FUNCTION FC 100 : VOID
TITLE =GESTIONE OUTPUT
AUTHOR : MassimoZ
VERSION : 0.1

BEGIN
NETWORK
TITLE =Spia Manuale
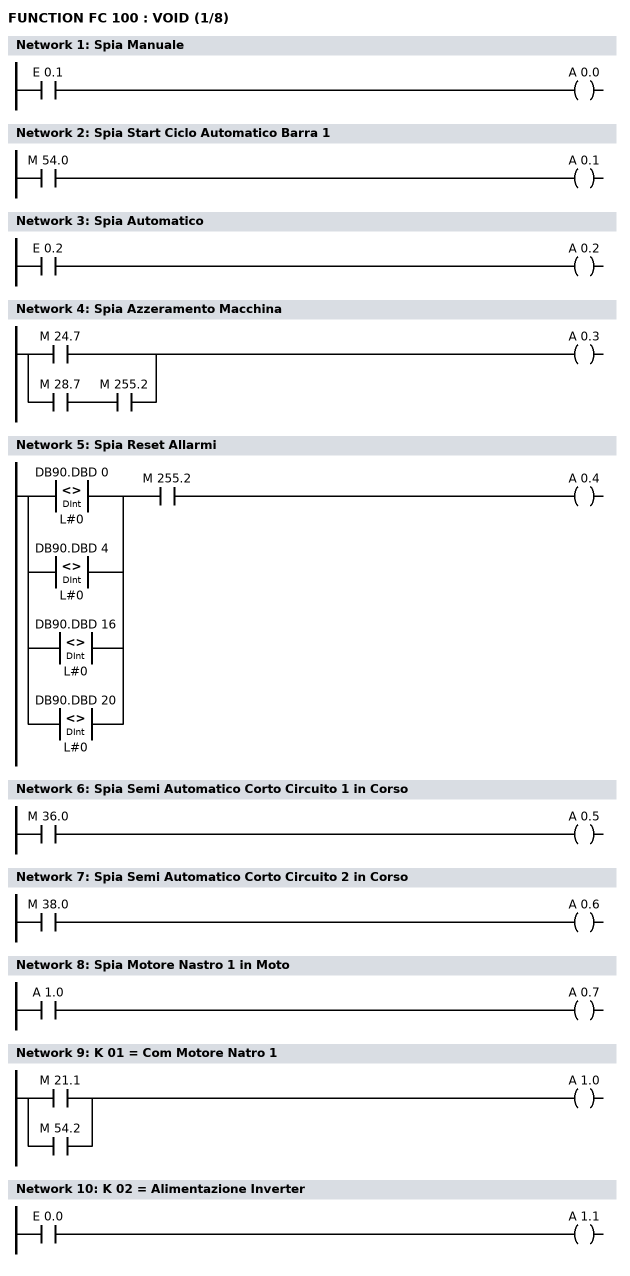
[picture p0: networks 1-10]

      U     E      0.1;
      =     A      0.0;
NETWORK
TITLE =Spia Start Ciclo Automatico Barra 1

      U     M     54.0;
      =     A      0.1;
NETWORK
TITLE =Spia Automatico

      U     E      0.2;
      =     A      0.2;
NETWORK
TITLE =Spia Azzeramento Macchina

      O     M     24.7;
      O     ;
      U     M     28.7;
      U     M    255.2;
      =     A      0.3;
NETWORK
TITLE =Spia Reset Allarmi

      U(    ;
      O(    ;
      L     DB90.DBD    0;
      L     L#0;
      <>D   ;
      )     ;
      O(    ;
      L     DB90.DBD    4;
      L     L#0;
      <>D   ;
      )     ;
      O(    ;
      L     DB90.DBD   16;
      L     L#0;
      <>D   ;
      )     ;
      O(    ;
      L     DB90.DBD   20;
      L     L#0;
      <>D   ;
      )     ;
      )     ;
      U     M    255.2;
      =     A      0.4;
NETWORK
TITLE =Spia Semi Automatico Corto Circuito 1 in Corso

      U     M     36.0;
      =     A      0.5;
NETWORK
TITLE =Spia Semi Automatico Corto Circuito 2 in Corso

      U     M     38.0;
      =     A      0.6;
NETWORK
TITLE =Spia Motore Nastro 1 in Moto

      U     A      1.0;
      =     A      0.7;
NETWORK
TITLE =K 01 = Com Motore Natro 1

      O     M     21.1;
      O     M     54.2;
      =     A      1.0;
NETWORK
TITLE =K 02 = Alimentazione Inverter

      U     E      0.0;
      =     A      1.1;
NETWORK
TITLE =K 03 = Com Motore Natro 3
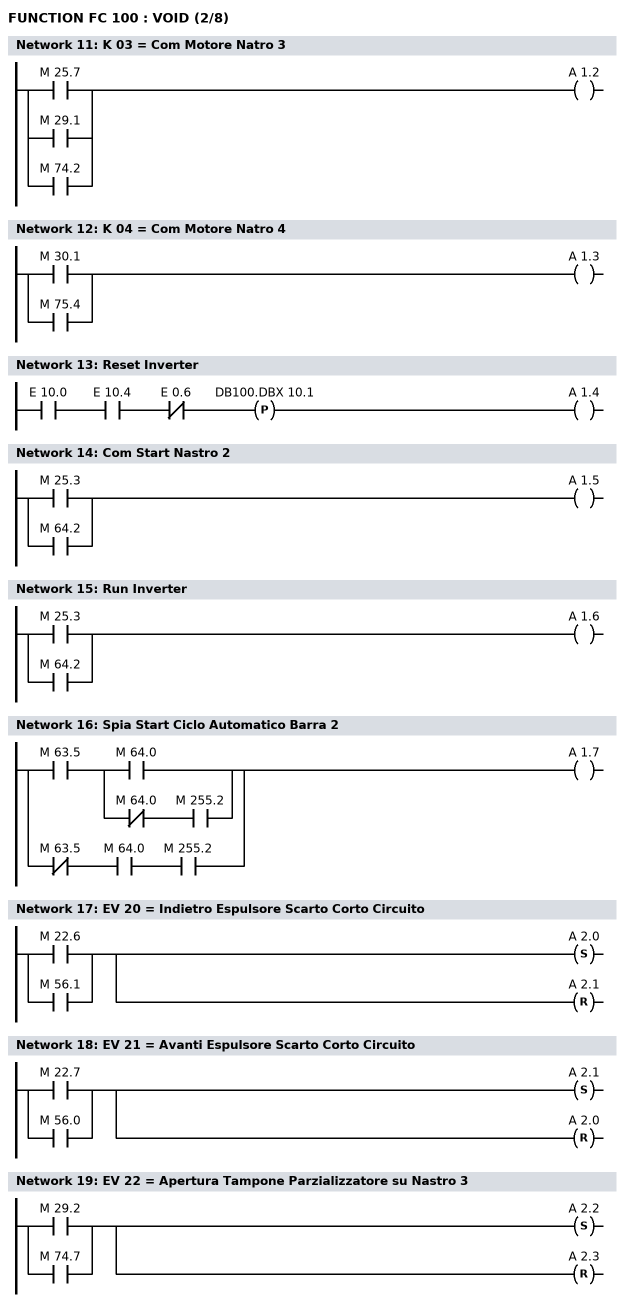
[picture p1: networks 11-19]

      O     M     25.7;
      O     M     29.1;
      O     M     74.2;
      =     A      1.2;
NETWORK
TITLE =K 04 = Com Motore Natro 4

      O     M     30.1;
      O     M     75.4;
      =     A      1.3;
NETWORK
TITLE =Reset Inverter

      U     E     10.0;
      U     E     10.4;
      UN    E      0.6;
      FP    DB100.DBX   10.1;
      =     A      1.4;
NETWORK
TITLE =Com Start Nastro 2

      O     M     25.3;
      O     M     64.2;
      =     A      1.5;
NETWORK
TITLE =Run Inverter

      O     M     25.3;
      O     M     64.2;
      =     A      1.6;
NETWORK
TITLE =Spia Start Ciclo Automatico Barra 2

      U     M     63.5;
      U(    ;
      O     M     64.0;
      O     ;
      UN    M     64.0;
      U     M    255.2;
      )     ;
      O     ;
      UN    M     63.5;
      U     M     64.0;
      U     M    255.2;
      =     A      1.7;
NETWORK
TITLE =EV 20 = Indietro Espulsore Scarto Corto Circuito

      O     M     22.6;
      O     M     56.1;
      S     A      2.0;
      R     A      2.1;
NETWORK
TITLE =EV 21 = Avanti Espulsore Scarto Corto Circuito

      O     M     22.7;
      O     M     56.0;
      S     A      2.1;
      R     A      2.0;
NETWORK
TITLE =EV 22 = Apertura Tampone Parzializzatore su Nastro 3

      O     M     29.2;
      O     M     74.7;
      S     A      2.2;
      R     A      2.3;
NETWORK
TITLE =EV 23 = Chiusura Tampone Parzializzatore su Nastro 3
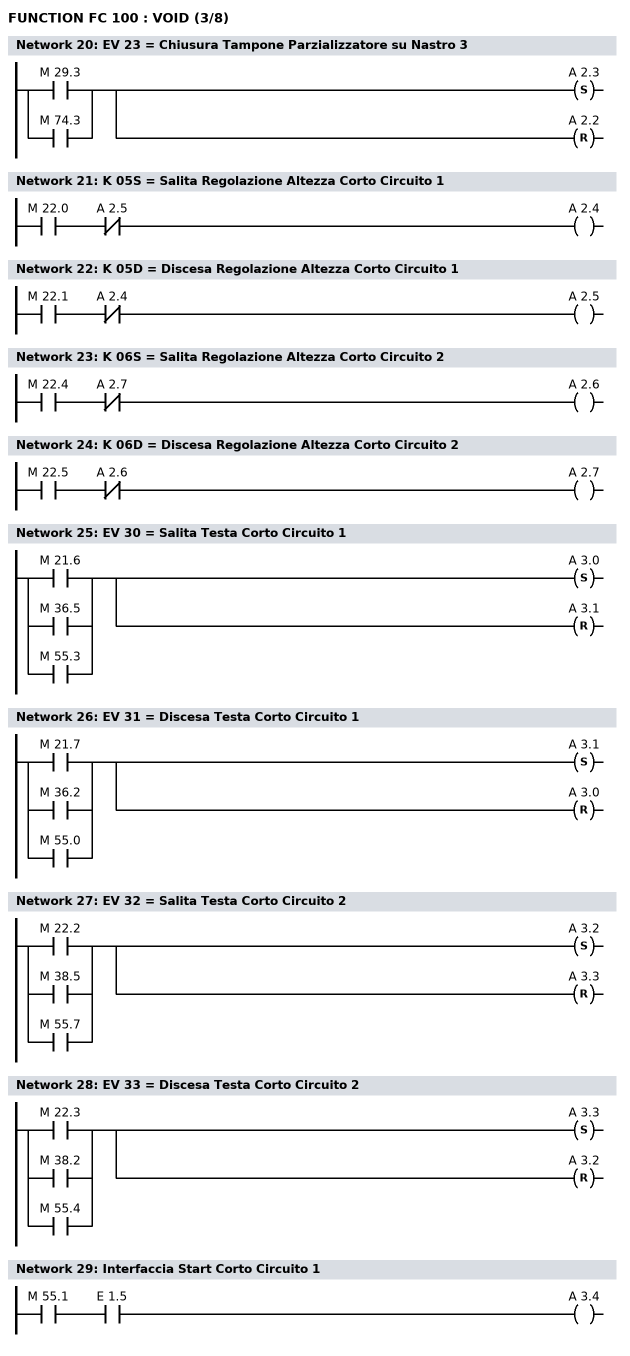
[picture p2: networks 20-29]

      O     M     29.3;
      O     M     74.3;
      S     A      2.3;
      R     A      2.2;
NETWORK
TITLE =K 05S = Salita Regolazione Altezza Corto Circuito 1

      U     M     22.0;
      UN    A      2.5;
      =     A      2.4;
NETWORK
TITLE =K 05D = Discesa Regolazione Altezza Corto Circuito 1

      U     M     22.1;
      UN    A      2.4;
      =     A      2.5;
NETWORK
TITLE =K 06S = Salita Regolazione Altezza Corto Circuito 2

      U     M     22.4;
      UN    A      2.7;
      =     A      2.6;
NETWORK
TITLE =K 06D = Discesa Regolazione Altezza Corto Circuito 2

      U     M     22.5;
      UN    A      2.6;
      =     A      2.7;
NETWORK
TITLE =EV 30 = Salita Testa Corto Circuito 1

      O     M     21.6;
      O     M     36.5;
      O     M     55.3;
      S     A      3.0;
      R     A      3.1;
NETWORK
TITLE =EV 31 = Discesa Testa Corto Circuito 1

      O     M     21.7;
      O     M     36.2;
      O     M     55.0;
      S     A      3.1;
      R     A      3.0;
NETWORK
TITLE =EV 32 = Salita Testa Corto Circuito 2

      O     M     22.2;
      O     M     38.5;
      O     M     55.7;
      S     A      3.2;
      R     A      3.3;
NETWORK
TITLE =EV 33 = Discesa Testa Corto Circuito 2

      O     M     22.3;
      O     M     38.2;
      O     M     55.4;
      S     A      3.3;
      R     A      3.2;
NETWORK
TITLE =Interfaccia Start Corto Circuito 1

      U     M     55.1;
      U     E      1.5;
      =     A      3.4;
NETWORK
TITLE =Interfaccia Start Corto Circuito 2
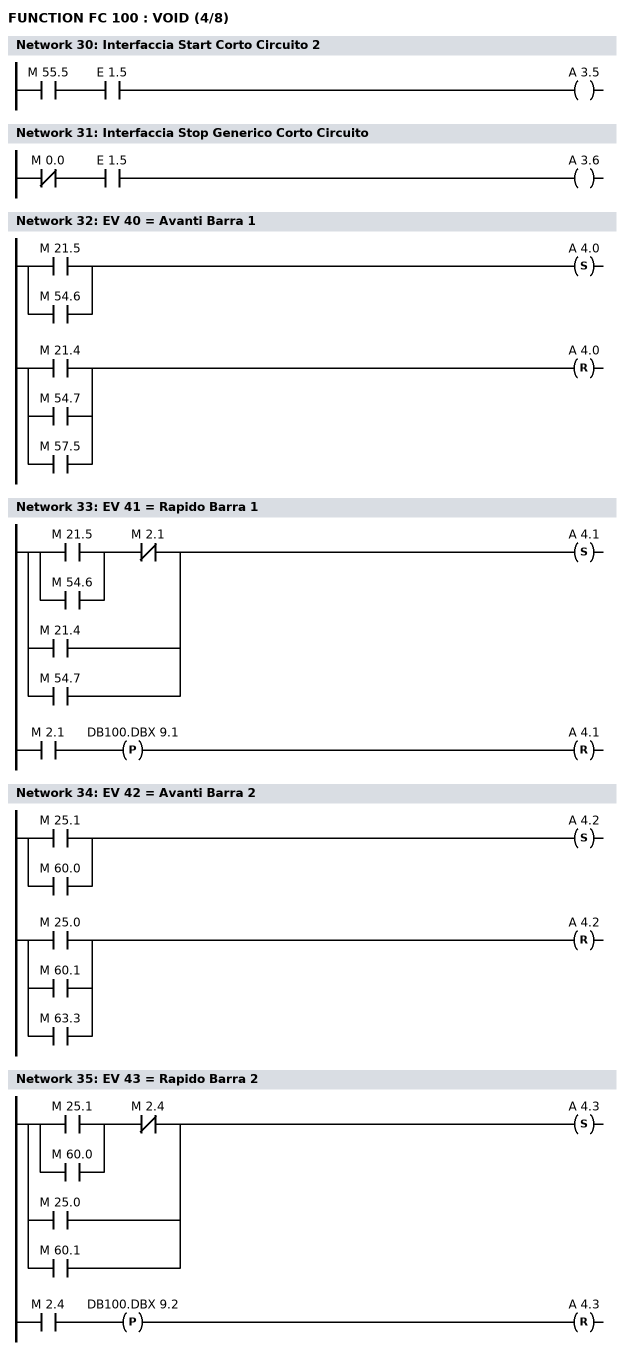
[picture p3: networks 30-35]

      U     M     55.5;
      U     E      1.5;
      =     A      3.5;
NETWORK
TITLE =Interfaccia Stop Generico Corto Circuito

      UN    M      0.0;
      U     E      1.5;
      =     A      3.6;
NETWORK
TITLE =EV 40 = Avanti Barra 1

      U(    ;
      O     M     21.5;
      O     M     54.6;
      )     ;
      S     A      4.0;
      U(    ;
      O     M     21.4;
      O     M     54.7;
      O     M     57.5;
      )     ;
      R     A      4.0;
      NOP   0;
NETWORK
TITLE =EV 41 = Rapido Barra 1

      U(    ;
      U(    ;
      O     M     21.5;
      O     M     54.6;
      )     ;
      UN    M      2.1;
      O     M     21.4;
      O     M     54.7;
      )     ;
      S     A      4.1;
      U     M      2.1;
      FP    DB100.DBX    9.1;
      R     A      4.1;
      NOP   0;
NETWORK
TITLE =EV 42 = Avanti Barra 2

      U(    ;
      O     M     25.1;
      O     M     60.0;
      )     ;
      S     A      4.2;
      U(    ;
      O     M     25.0;
      O     M     60.1;
      O     M     63.3;
      )     ;
      R     A      4.2;
      NOP   0;
NETWORK
TITLE =EV 43 = Rapido Barra 2

      U(    ;
      U(    ;
      O     M     25.1;
      O     M     60.0;
      )     ;
      UN    M      2.4;
      O     M     25.0;
      O     M     60.1;
      )     ;
      S     A      4.3;
      U     M      2.4;
      FP    DB100.DBX    9.2;
      R     A      4.3;
      NOP   0;
NETWORK
TITLE =EV 44 = Apertura Parzializzatore Inizio Linea
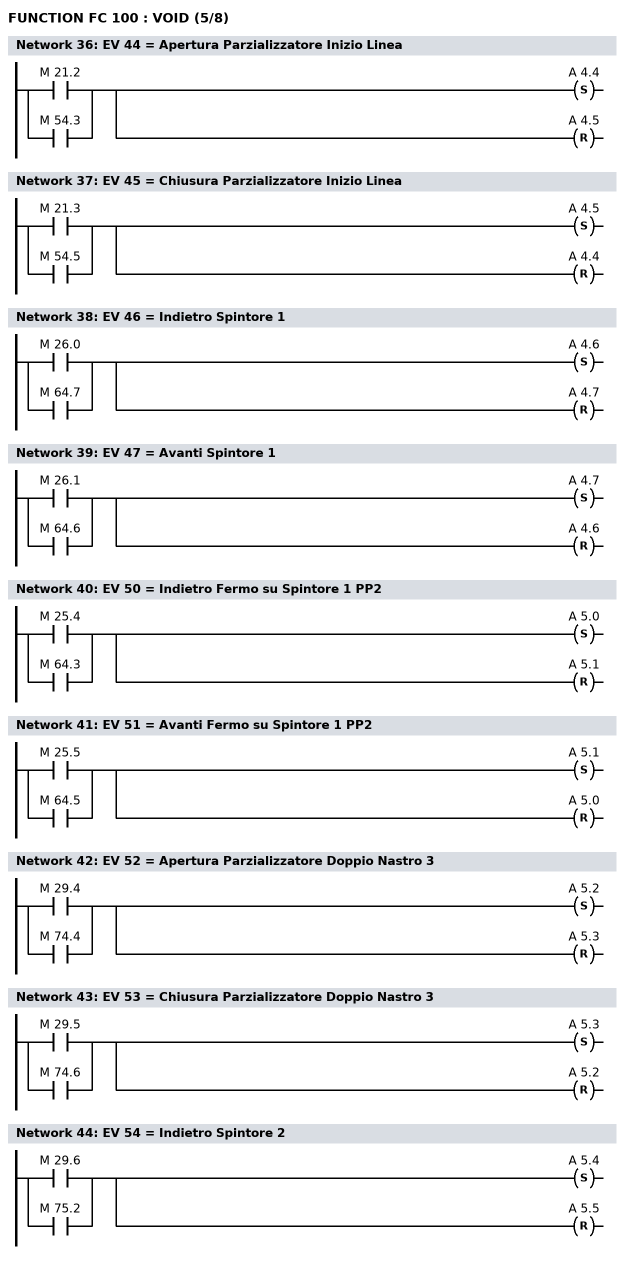
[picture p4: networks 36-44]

      O     M     21.2;
      O     M     54.3;
      S     A      4.4;
      R     A      4.5;
NETWORK
TITLE =EV 45 = Chiusura Parzializzatore Inizio Linea

      O     M     21.3;
      O     M     54.5;
      S     A      4.5;
      R     A      4.4;
NETWORK
TITLE =EV 46 = Indietro Spintore 1

      O     M     26.0;
      O     M     64.7;
      S     A      4.6;
      R     A      4.7;
NETWORK
TITLE =EV 47 = Avanti Spintore 1

      O     M     26.1;
      O     M     64.6;
      S     A      4.7;
      R     A      4.6;
NETWORK
TITLE =EV 50 = Indietro Fermo su Spintore 1 PP2

      O     M     25.4;
      O     M     64.3;
      S     A      5.0;
      R     A      5.1;
NETWORK
TITLE =EV 51 = Avanti Fermo su Spintore 1 PP2

      O     M     25.5;
      O     M     64.5;
      S     A      5.1;
      R     A      5.0;
NETWORK
TITLE =EV 52 = Apertura Parzializzatore Doppio Nastro 3

      O     M     29.4;
      O     M     74.4;
      S     A      5.2;
      R     A      5.3;
NETWORK
TITLE =EV 53 = Chiusura Parzializzatore Doppio Nastro 3

      O     M     29.5;
      O     M     74.6;
      S     A      5.3;
      R     A      5.2;
NETWORK
TITLE =EV 54 = Indietro Spintore 2

      O     M     29.6;
      O     M     75.2;
      S     A      5.4;
      R     A      5.5;
NETWORK
TITLE =EV 55 = Avanti Spintore 2
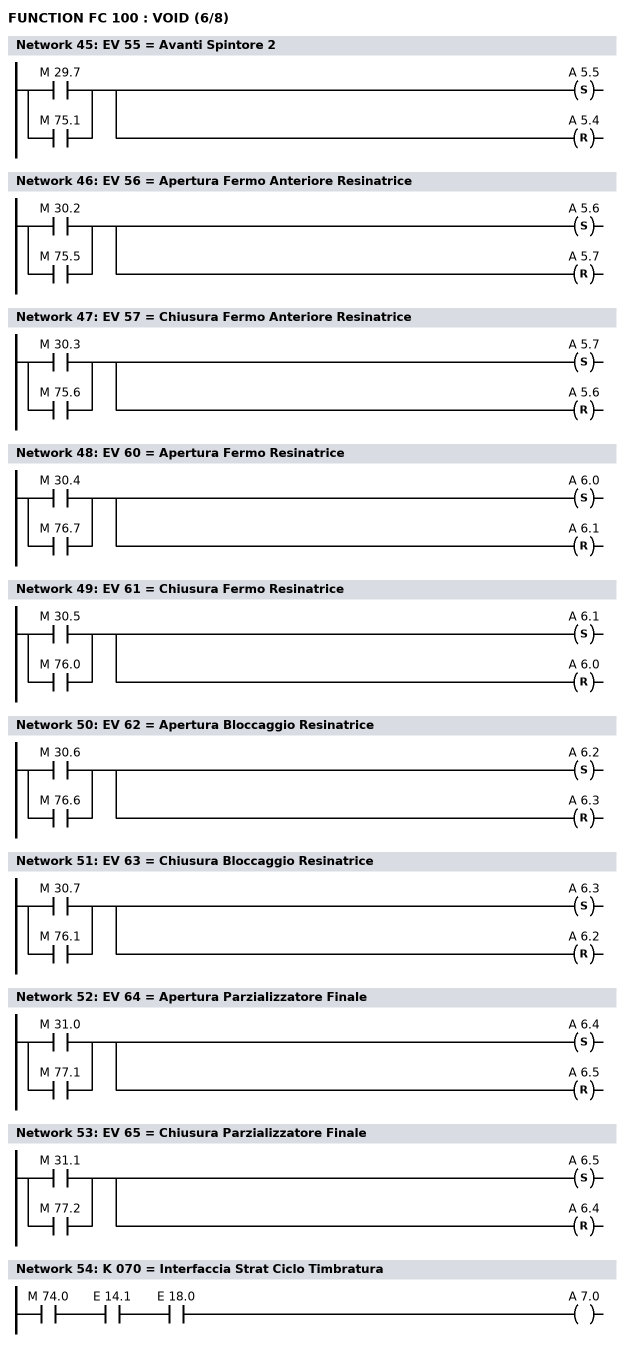
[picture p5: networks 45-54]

      O     M     29.7;
      O     M     75.1;
      S     A      5.5;
      R     A      5.4;
NETWORK
TITLE =EV 56 = Apertura Fermo Anteriore Resinatrice

      O     M     30.2;
      O     M     75.5;
      S     A      5.6;
      R     A      5.7;
NETWORK
TITLE =EV 57 = Chiusura Fermo Anteriore Resinatrice

      O     M     30.3;
      O     M     75.6;
      S     A      5.7;
      R     A      5.6;
NETWORK
TITLE =EV 60 = Apertura Fermo Resinatrice

      O     M     30.4;
      O     M     76.7;
      S     A      6.0;
      R     A      6.1;
NETWORK
TITLE =EV 61 = Chiusura Fermo Resinatrice

      O     M     30.5;
      O     M     76.0;
      S     A      6.1;
      R     A      6.0;
NETWORK
TITLE =EV 62 = Apertura Bloccaggio Resinatrice

      O     M     30.6;
      O     M     76.6;
      S     A      6.2;
      R     A      6.3;
NETWORK
TITLE =EV 63 = Chiusura Bloccaggio Resinatrice

      O     M     30.7;
      O     M     76.1;
      S     A      6.3;
      R     A      6.2;
NETWORK
TITLE =EV 64 = Apertura Parzializzatore Finale

      O     M     31.0;
      O     M     77.1;
      S     A      6.4;
      R     A      6.5;
NETWORK
TITLE =EV 65 = Chiusura Parzializzatore Finale

      O     M     31.1;
      O     M     77.2;
      S     A      6.5;
      R     A      6.4;
NETWORK
TITLE =K 070 = Interfaccia Strat Ciclo Timbratura

      U     M     74.0;
      U     E     14.1;
      U     E     18.0;
      =     A      7.0;
NETWORK
TITLE =K 071 = Interfaccia Strat Ciclo Resinatrice
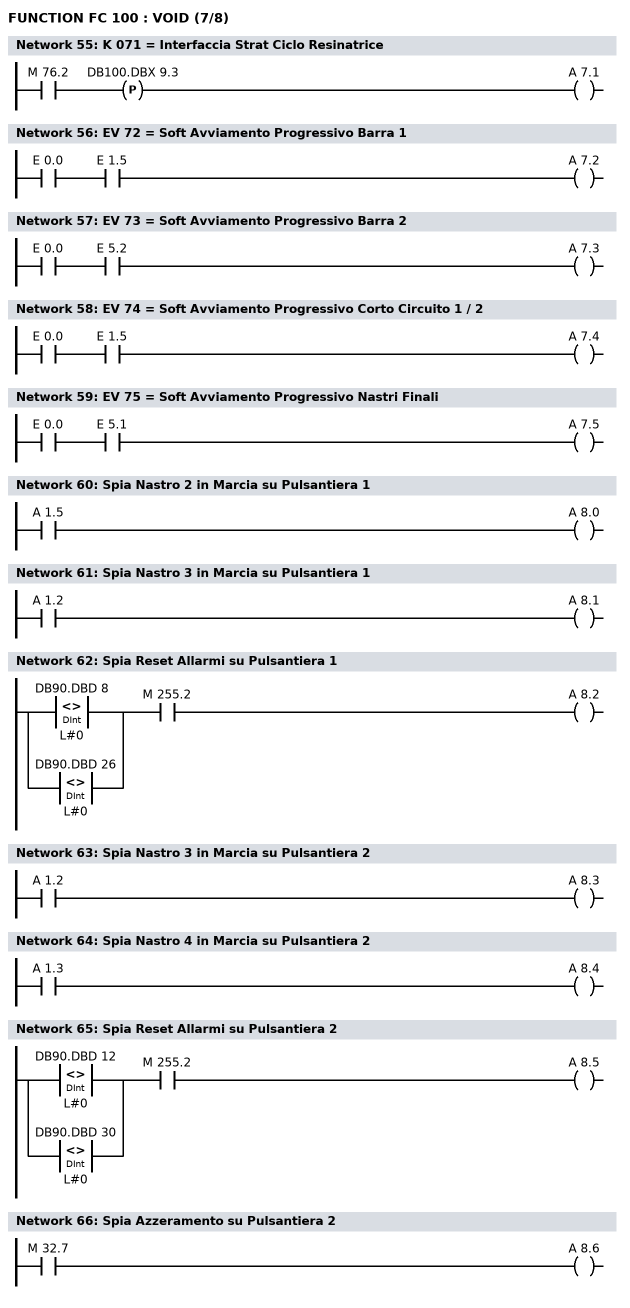
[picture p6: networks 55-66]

      U     M     76.2;
      FP    DB100.DBX    9.3;
      =     A      7.1;
NETWORK
TITLE =EV 72 = Soft Avviamento Progressivo Barra 1

      U     E      0.0;
      U     E      1.5;
      =     A      7.2;
NETWORK
TITLE =EV 73 = Soft Avviamento Progressivo Barra 2

      U     E      0.0;
      U     E      5.2;
      =     A      7.3;
NETWORK
TITLE =EV 74 = Soft Avviamento Progressivo Corto Circuito 1 / 2

      U     E      0.0;
      U     E      1.5;
      =     A      7.4;
NETWORK
TITLE =EV 75 = Soft Avviamento Progressivo Nastri Finali

      U     E      0.0;
      U     E      5.1;
      =     A      7.5;
NETWORK
TITLE =Spia Nastro 2 in Marcia su Pulsantiera 1

      U     A      1.5;
      =     A      8.0;
NETWORK
TITLE =Spia Nastro 3 in Marcia su Pulsantiera 1

      U     A      1.2;
      =     A      8.1;
NETWORK
TITLE =Spia Reset Allarmi su Pulsantiera 1

      U(    ;
      O(    ;
      L     DB90.DBD    8;
      L     L#0;
      <>D   ;
      )     ;
      O(    ;
      L     DB90.DBD   26;
      L     L#0;
      <>D   ;
      )     ;
      )     ;
      U     M    255.2;
      =     A      8.2;
NETWORK
TITLE =Spia Nastro 3 in Marcia su Pulsantiera 2

      U     A      1.2;
      =     A      8.3;
NETWORK
TITLE =Spia Nastro 4 in Marcia su Pulsantiera 2

      U     A      1.3;
      =     A      8.4;
NETWORK
TITLE =Spia Reset Allarmi su Pulsantiera 2

      U(    ;
      O(    ;
      L     DB90.DBD   12;
      L     L#0;
      <>D   ;
      )     ;
      O(    ;
      L     DB90.DBD   30;
      L     L#0;
      <>D   ;
      )     ;
      )     ;
      U     M    255.2;
      =     A      8.5;
NETWORK
TITLE =Spia Azzeramento su Pulsantiera 2

      U     M     32.7;
      =     A      8.6;
NETWORK
TITLE =Spia Start Lavorazione su Pulsantiera 2
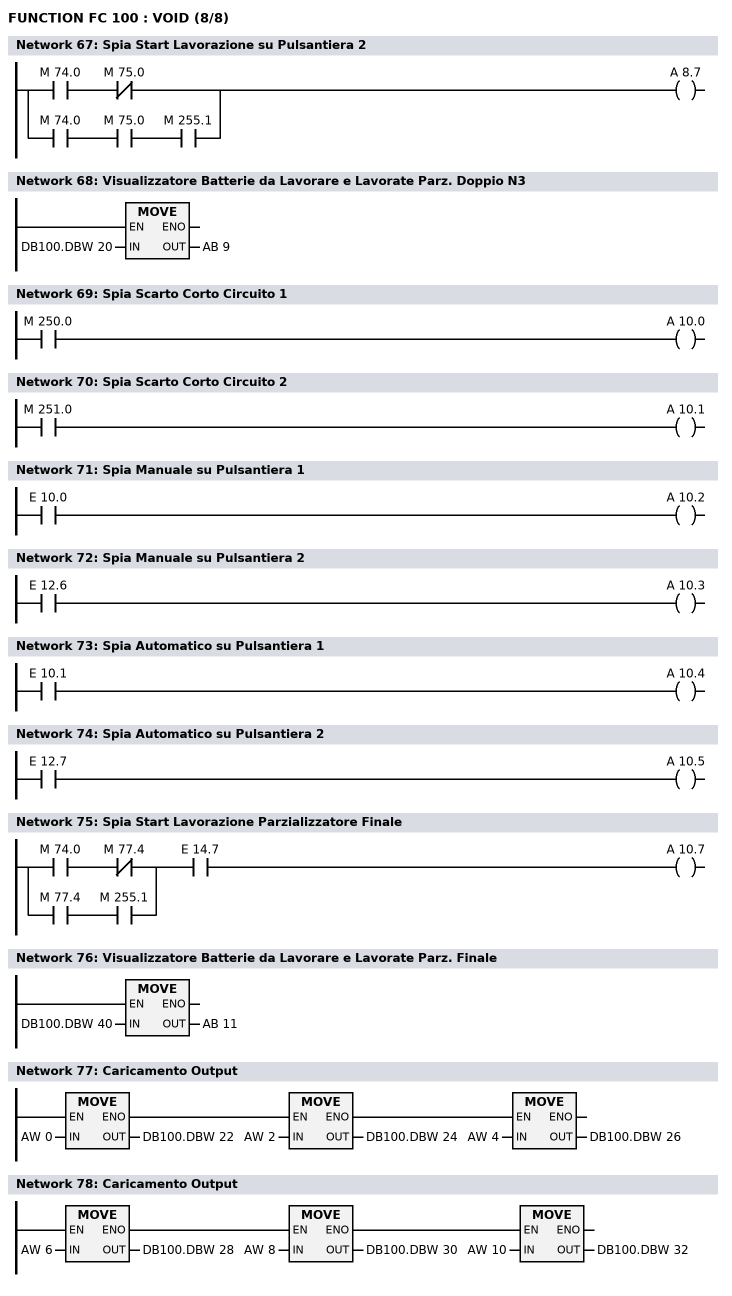
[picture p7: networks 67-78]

      U     M     74.0;
      UN    M     75.0;
      O     ;
      U     M     74.0;
      U     M     75.0;
      U     M    255.1;
      =     A      8.7;
NETWORK
TITLE =Visualizzatore Batterie da Lavorare e Lavorate Parz. Doppio N3


      L     DB100.DBW   20;
      T     AB     9;
      NOP   0;
NETWORK
TITLE =Spia Scarto Corto Circuito 1

      U     M    250.0;
      =     A     10.0;
NETWORK
TITLE =Spia Scarto Corto Circuito 2

      U     M    251.0;
      =     A     10.1;
NETWORK
TITLE =Spia Manuale su Pulsantiera 1

      U     E     10.0;
      =     A     10.2;
NETWORK
TITLE =Spia Manuale su Pulsantiera 2

      U     E     12.6;
      =     A     10.3;
NETWORK
TITLE =Spia Automatico su Pulsantiera 1

      U     E     10.1;
      =     A     10.4;
NETWORK
TITLE =Spia Automatico su Pulsantiera 2

      U     E     12.7;
      =     A     10.5;
NETWORK
TITLE =Spia Start Lavorazione Parzializzatore Finale

      U(    ;
      U     M     74.0;
      UN    M     77.4;
      O     ;
      U     M     77.4;
      U     M    255.1;
      )     ;
      U     E     14.7;
      =     A     10.7;
NETWORK
TITLE =Visualizzatore Batterie da Lavorare e Lavorate Parz. Finale

      L     DB100.DBW   40;
      T     AB    11;
      NOP   0;
NETWORK
TITLE =Caricamento Output

      U(    ;
      U(    ;
      L     AW     0;
      T     DB100.DBW   22;
      SET   ;
      SAVE  ;
      CLR   ;
      U     BIE;
      )     ;
      SPBNB _001;
      L     AW     2;
      T     DB100.DBW   24;
      SET   ;
      SAVE  ;
      CLR   ;
_001: U     BIE;
      )     ;
      SPBNB _002;
      L     AW     4;
      T     DB100.DBW   26;
_002: NOP   0;
NETWORK
TITLE =Caricamento Output

      U(    ;
      U(    ;
      L     AW     6;
      T     DB100.DBW   28;
      SET   ;
      SAVE  ;
      CLR   ;
      U     BIE;
      )     ;
      SPBNB _003;
      L     AW     8;
      T     DB100.DBW   30;
      SET   ;
      SAVE  ;
      CLR   ;
_003: U     BIE;
      )     ;
      SPBNB _004;
      L     AW    10;
      T     DB100.DBW   32;
_004: NOP   0;
END_FUNCTION

